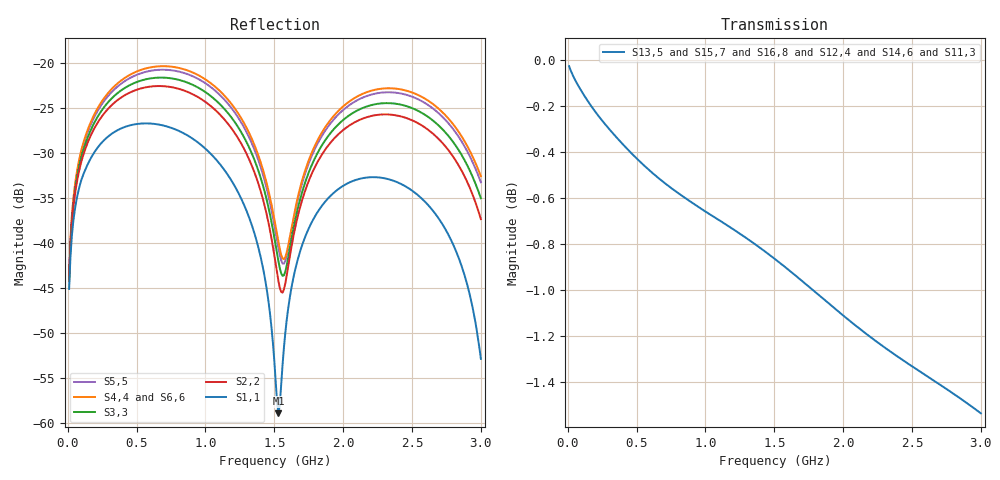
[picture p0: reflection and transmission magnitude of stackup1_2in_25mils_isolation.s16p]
! Touchstone file from project
# GHZ S RI R 50.000000
! Modal data exported
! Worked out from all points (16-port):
!   300 points, 10 MHz to 3 GHz, reference 50 ohm
!   strongest paths, dB at 10 MHz, 760 MHz, 1.51 GHz, 2.26 GHz, 3 GHz:
!     S13,5: 0.0, -0.6, -0.9, -1.2, -1.5
!     S15,7: 0.0, -0.6, -0.9, -1.2, -1.5
!     S16,8: 0.0, -0.6, -0.9, -1.2, -1.5
!     S12,4: 0.0, -0.6, -0.9, -1.2, -1.5
!     S14,6: 0.0, -0.6, -0.9, -1.2, -1.5
!     S11,3: 0.0, -0.6, -0.9, -1.2, -1.5
!   lowest |S11| = -58.9 dB at 1.53 GHz (marker M1), VSWR 1.00, Z = 50.1 - j0.0564 ohm
!   |S11| at or under -10 dB: start of sweep to end of sweep
